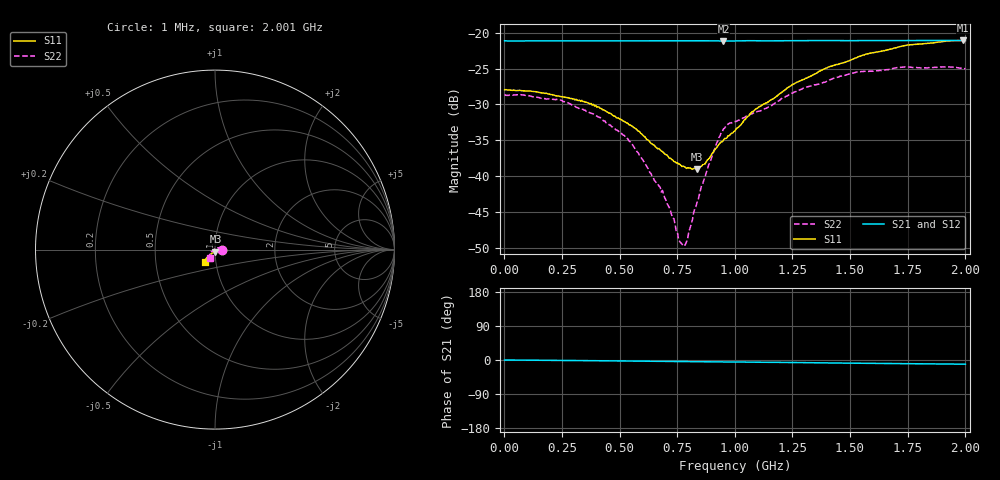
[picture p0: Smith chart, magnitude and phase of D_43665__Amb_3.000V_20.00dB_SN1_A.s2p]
! device id: 43665_
! dir: \\malibu\benchdata\1_engineers\tn_data\43665_75ohm\new\sparar\43665_\amb\3p000v\20p00db
! Serial: 1
! Insertion: A
! Temp: Amb
! VDD: 3.000V
! Attenuation Step: 20.00dB
! IDD: 1.453232e+00mA
! FILE NAME
! DATE 03-27-2009 08:38:15
! CORRECTED  DATA
#  Hz  S  RI  R  75
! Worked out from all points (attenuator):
!   401 points, 1 MHz to 2.001 GHz, reference 75 ohm
!   highest |S21| = -21.06 dB at 1.991 GHz (marker M1); lowest = -21.1 dB at 951 MHz (marker M2)
!   lowest |S11| = -39.1 dB at 836 MHz (marker M3), VSWR 1.02, Z = 75.4 - j1.64 ohm
!   |S11| at or under -10 dB: start of sweep to end of sweep
!   |S22| runs from -49.8 to -24.7 dB; largest |S21 - S12| = 0.0004
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1000000  0.0401 -0.000194  0.0881 -0.000102  0.0881 -0.000141  0.0371 -0.000196
2.36e8  0.0362 -0.000573  0.0879 -0.00166  0.0879 -0.00162  0.033 0.00803
3.36e8  0.0337 -0.00144  0.0879 -0.00243  0.0879 -0.00236  0.0274 0.0103
4.16e8  0.0297 -0.0015  0.0879 -0.00297  0.0879 -0.00294  0.0233 0.0106
5.31e8  0.0232 -0.00334  0.0879 -0.00401  0.0879 -0.00388  0.016 0.0093
6.71e8  0.0141 -0.00666  0.0879 -0.00511  0.0879 -0.00498  0.00578 0.00625
7.26e8  0.0105 -0.00782  0.0879 -0.00559  0.088 -0.00542  0.00207 0.00493
7.56e8  0.00842 -0.00873  0.0879 -0.00586  0.088 -0.00575  -0.000634 0.00355
7.76e8  0.00706 -0.00937  0.0879 -0.00611  0.0879 -0.00591  -0.002 0.00258
7.91e8  0.00578 -0.00972  0.0879 -0.00627  0.088 -0.0061  -0.00327 0.00119
8.36e8  0.00253 -0.0109  0.0879 -0.00672  0.0879 -0.00654  -0.00613 -0.00222
8.81e8  -0.00135 -0.0129  0.0877 -0.00722  0.0878 -0.00703  -0.0092 -0.00613
9.11e8  -0.00397 -0.0145  0.0875 -0.00755  0.0876 -0.00732  -0.0124 -0.00867
9.51e8  -0.00703 -0.0164  0.0873 -0.00771  0.0874 -0.00746  -0.0186 -0.0104
1.001e9  -0.0109 -0.0176  0.0875 -0.00776  0.0876 -0.00755  -0.0222 -0.0091
1.096e9  -0.0194 -0.0224  0.0876 -0.009  0.0877 -0.00872  -0.0239 -0.0149
1.251e9  -0.0307 -0.0309  0.0876 -0.0102  0.0878 -0.00996  -0.0279 -0.0257
1.336e9  -0.0359 -0.0355  0.0877 -0.011  0.0879 -0.0108  -0.0303 -0.0303
1.526e9  -0.0474 -0.0473  0.0873 -0.0129  0.0876 -0.0128  -0.0329 -0.0416
1.671e9  -0.0526 -0.0558  0.0872 -0.0143  0.0874 -0.0142  -0.0322 -0.0455
1.991e9  -0.0559 -0.0684  0.0869 -0.0169  0.087 -0.017  -0.0279 -0.0491
2.001e9  -0.0558 -0.0682  0.0868 -0.0169  0.0869 -0.017  -0.0279 -0.0487
